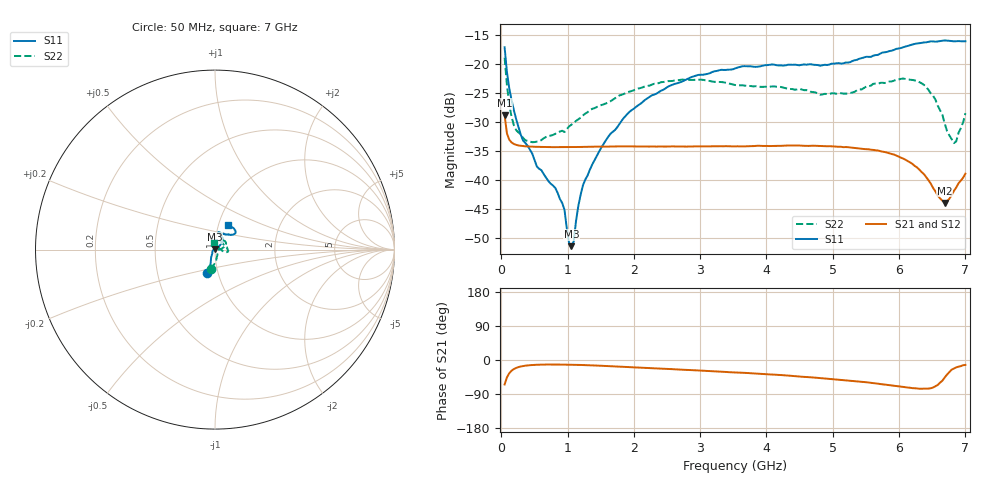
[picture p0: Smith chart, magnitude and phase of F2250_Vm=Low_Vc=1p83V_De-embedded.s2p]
! Integrated Device Technology
! Corporate Headquarters
! 6024 Silver Creek Valley Road
! San Jose, CA 95138  USA
! Phone:  1-408-284-8200
! Toll Free:  1-800-223-1366
! Webpage:  http://www.idt.com/
! Timing and RF Division
! 515 Groton Road, Suite 102
! Westford, MA 01886-6024
! Device:  F2250
! Description: Voltage Variable RF Attenuator
! Frequency:  50.0 -  6000.00 MHz
! Package:  3x3 mm Thin QFN Plastic Package: 16 pin
! Ports:  2 RF, 3 DC
!  Pin  1  = GND
!  Pin  2  = NC
!  Pin  3  = RF1  = Port 1
!  Pin  4  = NC
!  Pin  5  = GND
!  Pin  6  = GND
!  Pin  7  = GND
!  Pin  8  = GND
!  Pin  9  = NC
!  Pin 10  = RF2  = Port 2
!  Pin 11  = NC
!  Pin 12  = GND
!  Pin 13  = GND
!  Pin 14  = VCNTRL
!  Pin 15  = VDD
!  Pin 16  = VMODE
! Vcntrl:  1.830 Volts
! Vmode:  +0.000 Volts
! Vdd:  +3.30  Volts
! Current:  1.185 mA
! Data:  The device was measured on a the F2250 evaluation board which has
!  individual transmission lines to the RF pins.  Data was collected
!  using a calibrated network analyzer.  The evaluation board was
!  de-embedded using a TRL calibration technique.
!  The reference plane is the edge of the package pin.
! Misc:  SN 10
!  Action Tracker AT0258
! Date Measured:  2014-11-26
! Date:  2015-10-15  MJV
! Note:
!  Integrated Device Technology supplies this data as a sample of measured
!  data at the package pin for this product.  Your particular data for this
!  product may vary.
!  Data was taken at 25 degrees C.
!  Integrated Device Technology reserves the right to change this data at anytime.
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# GHz S dB R 50
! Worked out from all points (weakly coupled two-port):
!   201 points, 50 MHz to 7 GHz, reference 50 ohm
!   highest |S21| = -28.89 dB at 50 MHz (marker M1); lowest = -44.0 dB at 6.687 GHz (marker M2)
!   lowest |S11| = -51.5 dB at 1.058 GHz (marker M3), VSWR 1.01, Z = 49.9 + j0.235 ohm
!   |S11| at or under -10 dB: start of sweep to end of sweep
!   |S22| runs from -33.7 to -19.0 dB; largest |S21 - S12| = 6.3e-05
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0.05  -17.17 -108.4  -28.89 -64.6  -28.89 -64.6  -18.97 -101.1
0.08475  -21.43 -107.1  -32.00 -45.9  -32.00 -45.9  -23.70 -85.5
0.15425  -26.24 -116.2  -33.58 -28.3  -33.58 -28.3  -29.15 -70.4
0.36275  -33.66 -138.4  -34.25 -15.0  -34.24 -15.0  -33.21 -26.1
0.91875  -44.03 157.9  -34.40 -12.1  -34.39 -12.1  -31.56 1.2
0.9535  -45.20 169.9  -34.39 -12.2  -34.39 -12.2  -31.78 3.6
1.023  -50.96 142.2  -34.39 -12.4  -34.39 -12.4  -30.80 6.2
1.05775  -51.46 118.3  -34.39 -12.5  -34.39 -12.5  -30.52 7.2
1.0925  -50.63 83.8  -34.38 -12.6  -34.38 -12.6  -30.24 7.0
1.162  -44.52 53.7  -34.36 -12.9  -34.37 -12.9  -29.59 6.3
1.2315  -40.97 42.2  -34.34 -13.3  -34.34 -13.2  -28.94 5.7
1.6485  -32.07 41.2  -34.29 -16.2  -34.29 -16.2  -26.48 14.7
2.37825  -24.88 47.0  -34.28 -22.5  -34.28 -22.5  -23.34 25.3
3.525  -20.82 72.3  -34.27 -32.7  -34.26 -32.7  -23.68 53.0
4.7065  -20.19 72.3  -34.14 -46.2  -34.14 -46.3  -24.91 58.2
5.22775  -19.81 56.2  -34.39 -54.3  -34.39 -54.3  -25.14 34.1
5.85325  -17.83 40.4  -35.46 -66.4  -35.46 -66.4  -23.07 2.0
6.3745  -16.34 41.3  -39.04 -75.9  -39.07 -75.9  -23.65 -12.5
6.54825  -16.20 45.0  -42.03 -69.3  -42.07 -69.2  -26.20 -12.9
6.68725  -16.00 48.7  -44.02 -46.3  -44.02 -45.9  -30.27 4.8
6.82625  -16.15 53.5  -41.96 -22.5  -41.93 -22.4  -33.70 49.5
7  -16.13 63.2  -38.96 -13.0  -38.92 -13.1  -28.53 101.6
